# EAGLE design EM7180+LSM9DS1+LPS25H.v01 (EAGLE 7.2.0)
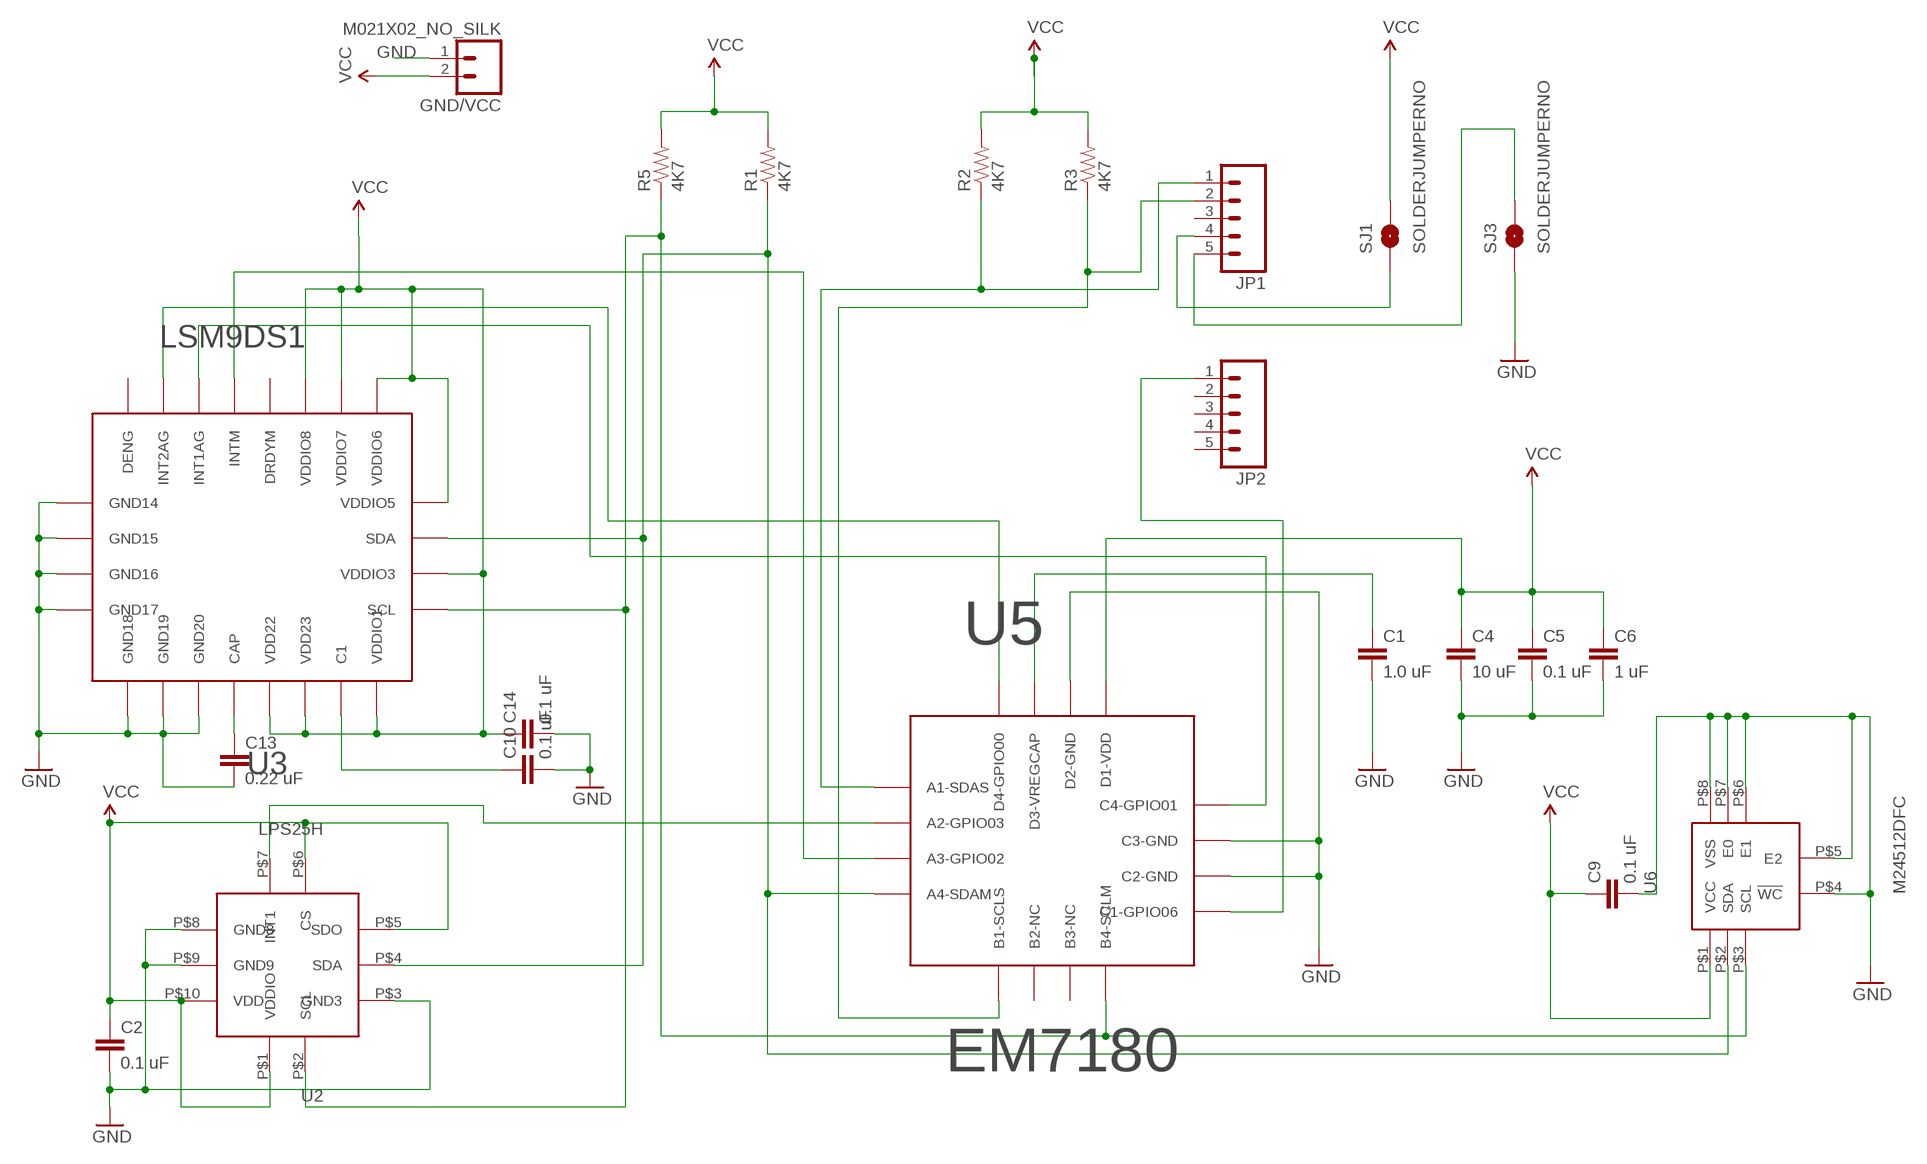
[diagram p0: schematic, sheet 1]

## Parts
C1  1.0 uF  CAP0402-CAP  [0402-CAP]
C2  0.1 uF  CAP0402-CAP  [0402-CAP]
C4  10 uF  CAP0402-CAP  [0402-CAP]
C5  0.1 uF  CAP0402-CAP  [0402-CAP]
C6  1 uF  CAP0402-CAP  [0402-CAP]
C9  0.1 uF  CAP0402-CAP  [0402-CAP]
C10  0.1 uF  CAP0402-CAP  [0402-CAP]
C13  0.22 uF  CAP0402-CAP  [0402-CAP]
C14  0.1 uF  CAP0402-CAP  [0402-CAP]
GND/VCC  M021X02_NO_SILK  [1X02_NO_SILK]
JP1  M05NO_SILK  [1X05_NO_SILK]
JP2  M05NO_SILK  [1X05_NO_SILK]
R1  4K7  0402RES.KW  [0402-RES]
R2  4K7  0402RES.KW  [0402-RES]
R3  4K7  0402RES.KW  [0402-RES]
R5  4K7  0402RES.KW  [0402-RES]
SJ1  SOLDERJUMPERNO  [SJ_2S-NO]
SJ3  SOLDERJUMPERNO  [SJ_2S-NO]
U2  LPS25H  [HCLGA-10L]
U3  LSM9DS1  [LGA-24LONG]
U5  EM7180  [WL-CSP16]
U6  M24512DFC  [M24512DFC]

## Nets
GND: C1.2 C2.2 C4.2 C5.2 C6.2 C9.2 C10.2 C13.2 C14.2 GND/VCC.1 SJ3.1 U2.P$3(GND3) U2.P$8(GND8) U2.P$9(GND9) U3.P$14(GND14) U3.P$15(GND15) U3.P$16(GND16) U3.P$17(GND17) U3.P$18(GND18) U3.P$19(GND19) U3.P$20(GND20) U5.P$10(C2-GND) U5.P$11(C3-GND) U5.P$14(D2-GND) U6.P$4(!WC) U6.P$5(E2) U6.P$6(E1) U6.P$7(E0) U6.P$8(VSS)
N$1: U2.P$7(INT1) U5.P$2(A2-GPIO03)
N$2: U3.P$10(INTM) U5.P$3(A3-GPIO02)
N$4: JP2.1 U5.P$9(C1-GPIO06)
N$5: U3.P$11(INT1AG) U5.P$12(C4-GPIO01)
N$6: U3.P$12(INT2AG) U5.P$16(D4-GPIO00)
N$7: JP1.4 SJ1.1
N$8: JP1.5 SJ3.2
N$9: C1.1 U5.P$15(D3-VREGCAP)
N$12: C13.1 U3.P$21(CAP)
N$14: C10.1 U3.P$24(C1)
SCL: R5.1 U2.P$2(SCL) U3.P$2(SCL) U5.P$8(B4-SCLM) U6.P$3(SCL)
SCL1: JP1.1 R2.1 U5.P$1(A1-SDAS)
SDA: R1.1 U2.P$4(SDA) U3.P$4(SDA) U5.P$4(A4-SDAM) U6.P$2(SDA)
SDA1: JP1.2 R3.1 U5.P$5(B1-SCLS)
VCC: C2.1 C4.1 C5.1 C6.1 C9.1 C14.1 GND/VCC.2 R1.2 R2.2 R3.2 R5.2 SJ1.2 U2.P$1(VDDIO) U2.P$5(SDO) U2.P$6(CS) U2.P$10(VDD) U3.P$1(VDDIO1) U3.P$3(VDDIO3) U3.P$5(VDDIO5) U3.P$6(VDDIO6) U3.P$7(VDDIO7) U3.P$8(VDDIO8) U3.P$22(VDD22) U3.P$23(VDD23) U5.P$13(D1-VDD) U6.P$1(VCC)
Unconnected: JP1.3 JP2.2 JP2.3 JP2.4 JP2.5 U3.P$9(DRDYM) U3.P$13(DENG) U5.P$6(B2-NC) U5.P$7(B3-NC)

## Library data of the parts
C1 C2 C4-C6 C9 C10 C13 C14 = SparkFun-Capacitors:CAP: Capacitor
GND/VCC = SparkFun-Connectors:M02: Standard 2-pin 0.1" header. Use with
JP1 JP2 = SparkFun-Connectors:M05: Header 5 Standard 5-pin 0.1" header. Use with straight break away headers (SKU : PRT-00116), right angle break away headers (PRT-00553), swiss pins (PRT-00743), machine pins (PRT-00117), and female headers (PRT-00115). Molex polarized connector foot print use with SKU : PRT-08230 with associated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
R1-R3 R5 = SparkFun-Resistors:0402RES.KW
SJ1 SJ3 = SparkFun-Retired:SOLDERJUMPER: Solder Jumper
U2 = Kris:LPS25H: HCLGA-10L package for the LPS25H ST pressure sensor
U3 = SparkFun-DigitalIC:LSM9DS1: LSM9DS1 3.0 mm x 3.5 mm 9-axis motion sensor by ST Microelectrinics in an LGA-24 device package
U5 = SparkFun-DigitalIC:EM7180: WL-CSP19 package for the EM7180 SENtral sensor fusion hub
U6 = Kris:M24512DFC: ST's M24512DFC6 512 Mbit EEPROM

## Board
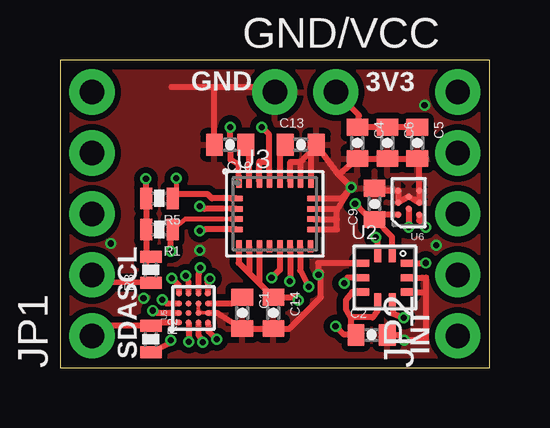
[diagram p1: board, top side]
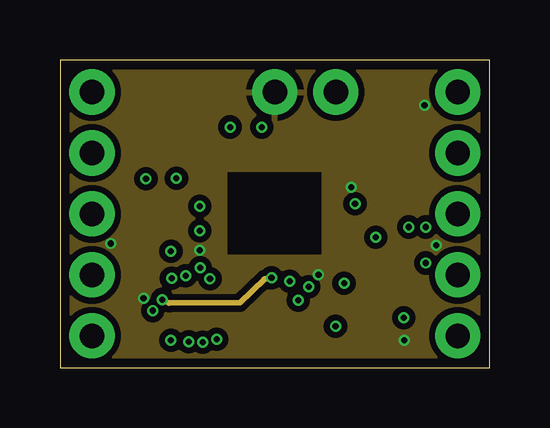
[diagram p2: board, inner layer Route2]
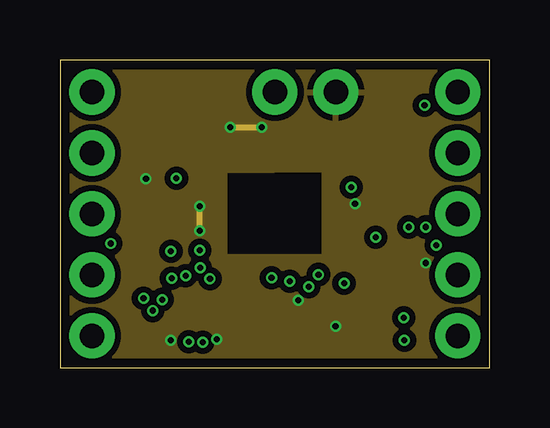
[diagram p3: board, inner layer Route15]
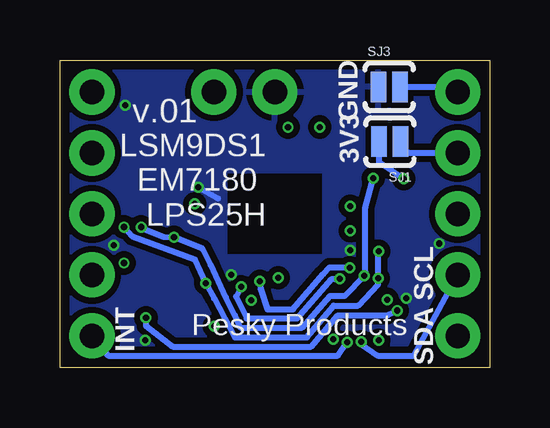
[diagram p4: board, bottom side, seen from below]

Size 17.91 x 12.83 mm. Coordinates in mm from the lower left corner, seen from the top.
Outline: 0,0 17.91,0 17.91,12.83 0,12.83 0,0
Copper layers (1*2*15*16): Top 0.035559375mm / dielectric 0.17018125mm / Route2 0.01778125mm / dielectric 47mil / Route15 0.01778125mm / dielectric 0.17018125mm / Bottom 0.035559375mm
Design rules "OSHPark-4layer *": minimum track width 5mil, minimum drill 10mil, track to track 5mil, track to pad 5mil, pad to pad 5mil, via to via 5mil, smd to smd 5mil, copper to edge 15mil, drill to drill 6mil, minimum pad ring 4mil, minimum via ring 4mil, stop-mask expansion 4mil, vias tented up to drill 20mil, thermal gap 10mil

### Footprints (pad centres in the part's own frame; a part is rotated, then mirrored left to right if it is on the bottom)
0402-CAP = smd 0.7 x 0.9: 1 -0.65,0; 2 0.65,0
1X02_NO_SILK = drill 1.016 pad 1.88: 1 0,0; 2 2.54,0
1X05_NO_SILK = drill 1.016 pad 1.88: 1 0,0; 2 2.54,0; 3 5.08,0; 4 7.62,0; 5 10.16,0
0402-RES = smd 0.5 x 0.9: 1 -0.55,0; 2 0.55,0
SJ_2S-NO = smd 0.635 x 1.27: 1 -0.45,0; 2 0.45,0
HCLGA-10L = smd 0.3 x 0.6: P$1 0.3,0.95; P$2 -0.3,0.95; P$6 -0.3,-0.95; P$7 0.3,-0.95 | smd 0.6 x 0.3: P$3 -0.95,0.6; P$4 -0.95,0; P$5 -0.95,-0.6; P$8 0.95,-0.6; P$9 0.95,0; P$10 0.95,0.6
LGA-24LONG = smd 0.23 x 0.5: P$1 -1.505,1.345; P$6 -1.505,-1.345; P$7 -1.075,-1.345; P$8 -0.645,-1.345; P$9 -0.22,-1.345; P$10 0.205,-1.345; P$11 0.63,-1.345; P$12 1.055,-1.345; P$13 1.48,-1.345; P$18 1.505,1.345; P$19 1.075,1.345; P$20 0.645,1.345; P$21 0.215,1.345; P$22 -0.215,1.345; P$23 -0.645,1.345; P$24 -1.075,1.345 | smd 0.5 x 0.23: P$2 -1.595,0.645; P$3 -1.595,0.215; P$4 -1.595,-0.215; P$5 -1.595,-0.645; P$14 1.595,-0.645; P$15 1.595,-0.215; P$16 1.595,0.215; P$17 1.595,0.645
WL-CSP16 = smd 0.24 x 0.24: P$1 -0.6,0.6; P$2 -0.2,0.6; P$3 0.2,0.6; P$4 0.6,0.6; P$5 -0.6,0.2; P$6 -0.2,0.2; P$7 0.2,0.2; P$8 0.6,0.2; P$9 -0.6,-0.2; P$10 -0.2,-0.2; P$11 0.2,-0.2; P$12 0.6,-0.2; P$13 -0.6,-0.6; P$14 -0.2,-0.6; P$15 0.2,-0.6; P$16 0.6,-0.6
M24512DFC = smd 0.27 x 0.27: P$1 0.433,0.5; P$2 -0.433,0.5; P$3 0,0.25; P$4 0.433,0; P$5 -0.433,0; P$6 0,-0.25; P$7 0.433,-0.5; P$8 -0.433,-0.5

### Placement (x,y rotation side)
C1  7.59,2.29 270 top
C2  12.98,1.37 0 top
C4  12.39,9.37 270 top
C5  14.88,9.37 270 top
C6  13.64,9.37 270 top
C9  13.11,6.83 90 top
C10  7.09,9.3 180 top
C13  10.03,9.3 0 top
C14  8.89,2.29 270 top
GND/VCC  8.95,11.49 0 top
JP1  1.33,1.33 90 top
JP2  16.57,1.33 90 top
R1  4.14,5.77 180 top
R2  3.78,1.19 270 top
R3  3.78,4.09 90 top
R5  4.14,7.06 180 top
SJ1  4.17,9.42 180 bottom
SJ3  4.19,11.71 0 bottom
U2  13.54,3.76 0 top
U3  8.95,6.41 0 top
U5  5.56,2.49 90 top
U6  14.53,6.88 180 top

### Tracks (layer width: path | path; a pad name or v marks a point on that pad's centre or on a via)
GND  (via drill 0.25)
  Top 0.152: U5.P$11 U5.P$10 U5.P$14
  Top 0.254: SJ3.1 6.38,11.71 | 6.38,11.71 8.74,11.71 GND/VCC.1 | U5.P$14 6.56,2.29 C1.2 C14.2 9.56,1.64 10.87,2.95 10.87,3.99 v10.77,3.89 10.76,4.36 U2.P$3 | U3.P$19 10.03,8.59 | 10.03,8.59 C13.2 | U3.P$20 9.6,8.13 9.6,8.59 10.03,8.59 | C2.2 14.07,1.37 v14.35,1.14 15.16,1.14 15.24,1.22 15.24,3.12 | U3.P$17 11.76,7.06 v12.14,7.52 | U3.P$14 11.53,5.77 11.53,6.17 | 11.53,6.17 11.53,6.55 | 11.53,6.55 12.09,7.47 v12.14,7.52 | U3.P$16 11.46,6.63 11.53,6.55 | U3.P$15 11.51,6.2 11.53,6.17 | U3.P$18 10.46,8.89 C13.2 | v12.14,7.52 11.58,8.09 | 11.58,8.09 C13.2 | 11.58,8.09 11.66,8.09 C4.2 C6.2 C5.2 14.96,8.85 U6.P$8 U6.P$5 14.76,7.01 U6.P$6 14.32,7.01 U6.P$4 U6.P$7 13.21,7.38 C9.2 | U2.P$9 15.24,3.76 15.24,3.12 | U2.P$8 15.21,3.16 15.24,3.12 | C10.2 6.44,11.65 6.38,11.71
  Bottom 0.254: v12.14,7.52 11.33,7.06
  other vias: 15.19,10.95 2.11,5.18 5.82,4.9 15.67,5.11 3.48,2.9
  pour Bottom (isolate 0.254): 0,12.83 17.91,12.83 17.91,0 11,0 11,8.18 6.91,8.18 6.91,4.67 10.92,4.67 10.92,0 0.03,0
  pour Route2 (isolate 0.254): 0,12.83 17.91,12.83 17.91,0 10.97,0 10.97,8.2 6.91,8.23 6.91,4.67 10.87,4.65 10.87,0 0.03,0
  pour Top (isolate 0.254): 0,12.83 17.86,12.83 17.86,0 14.83,0 14.83,5.08 12.24,5.08 12.24,2.46 14.76,2.46 14.76,0 10.9,0 10.95,8.15 6.91,8.15 6.93,4.67 10.82,4.67 10.82,0 -0.03,0 -0.03,12.8
N$1  (via drill 0.25)
  Top 0.254: U2.P$7 13.86,2.27 v14.33,2.08 | v3.86,2.39 4.05,2.29 U5.P$2
  Bottom 0.254: v14.33,2.08 14.33,1.75 13.21,0.89 7.44,0.89 6.33,2.18 4.27,2.18 v3.86,2.39
N$2  (via drill 0.25)
  Top 0.254: U3.P$10 9.16,4.08 v8.81,3.76 | v4.27,2.85 4.41,2.69 U5.P$3
  Route2 0.254: v8.81,3.76 8.51,3.68 7.49,2.72 4.55,2.69 v4.27,2.85
N$4  (via drill 0.25)
  Top 0.254: U5.P$9 5.76,1.38 v5.94,1.07
  Bottom 0.254: JP2.1 15.9,0.51 6.33,0.51 v5.94,1.07
N$5  (via drill 0.25)
  Top 0.254: U3.P$11 9.58,3.64 v9.58,3.61 | v5.84,4.17 5.77,3.86 U5.P$12
  Bottom 0.254: v9.58,3.61 9.55,3.28 9.27,2.44 8.2,2.44 6.93,3.91 6.68,4.19 5.92,4.19 v5.84,4.17
N$6  (via drill 0.25)
  Top 0.254: U3.P$12 10.01,4.06 v10.36,3.38 | v6.25,3.71 6.15,3.56 6.15,3.1 U5.P$16
  Bottom 0.254: v10.36,3.38 10.57,2.97 10.13,2.06 8.03,2.06 6.58,3.71 v6.25,3.71
N$7
  Bottom 0.152: 3.76,9.04 SJ1.1
  Bottom 0.254: 3.76,9.04 3.79,9.09 3.38,8.97 1.88,8.97 JP1.4
N$8
  Bottom 0.254: 3.68,12.22 SJ3.2 1.55,11.71 JP1.5
N$9
  Top 0.254: U5.P$15 7.15,2.69 C1.1
N$12
  Top 0.254: U3.P$21 9.17,9 C13.1
N$14
  Top 0.254: U3.P$24 7.88,8.9 C10.1
SCL  (via drill 0.25)
  Top 0.203: v4.85,7.9 4.85,7.48 R5.1
  Top 0.254: U5.P$8 5.36,3.58 v5.23,3.83 | R5.1 4.87,7.24 6.15,7.24 6.33,7.06 U3.P$2 | U2.P$2 13.24,5.05 13.23,5.28 13.18,5.41 v13.16,5.44 | U6.P$3 v14.53,5.87
  Bottom 0.254: v4.85,7.9 5.18,6.68 5.18,3.99 v5.23,3.83 6.04,3 6.66,3 7.82,1.68 10.39,1.68 10.62,2.18 11,2.92 11.63,4.29 11.96,4.95 v13.16,5.44 13.59,5.46 14.38,5.77 v14.53,5.87
SCL1
  Top 0.254: JP1.1 1.79,1.74 R2.1 4.05,1.89 U5.P$1
SDA  (via drill 0.25)
  Top 0.203: U3.P$4 5.22,6.2 R1.1
  Top 0.254: U5.P$4 4.96,3.42 v4.65,3.73 | v4.62,4.85 4.62,5.6 R1.1 | U2.P$4 11.99,3.76 v11.84,3.53 | U6.P$2 14.96,6.15 v15.24,5.87
  Bottom 0.254: v4.62,4.85 4.65,4.62 v4.65,3.73 4.65,3.48 5.49,2.59 6.5,2.59 7.62,1.27 10.62,1.27 11.48,2.9 v11.84,3.53 12.29,4.52 14.9,5.49 v15.24,5.87
SDA1  (via drill 0.25)
  Top 0.254: R3.1 2.15,3.56 JP1.2 | U5.P$5 v5.36,1.09
  Bottom 0.254: v5.36,1.09 5.36,0.99 4.67,0.51 3.17,0.51 JP1.2
VCC  (via drill 0.25)
  Top 0.254: C5.1 C6.1 C4.1 12.46,10.52 GND/VCC.2 10.79,11.48 | U6.P$1 13.23,6.38 C9.1 | v3.58,7.87 3.58,7.59 R5.2 R1.2 3.59,4.35 R3.2 | R2.2 4.55,1.02 v4.62,1.14 | U5.P$13 6.19,1.51 v6.53,1.19 | C9.1 13.08,6.02 v12.29,6.83 | U3.P$6 7.45,4.38 | U2.P$1 13.84,5.45 C9.1 | U2.P$6 13.24,2.39 13.03,2.11 12.14,2.11 12.12,2.06 | U2.P$5 12.18,3.16 11.91,2.82 11.91,2.44 12.12,2.06 | U2.P$10 v15.23,4.36 v15.24,4.37 | v11.48,1.73 11.83,1.38 12.12,1.38 C2.1 12.12,1.58 12.12,2.06 | U3.P$22 8.71,8.63 | U3.P$23 8.31,8.59 8.67,8.59 8.71,8.63 | U3.P$1 7.45,8 7.44,8.46 7.11,8.66 v7.09,10.03 | U3.P$5 6.05,5.77 v5.82,5.71 | U3.P$7 7.88,3.95 | U3.P$8 8.31,3.52 | 7.45,4.38 7.88,3.95 | 7.44,4.37 7.45,4.38 | U3.P$3 6.02,6.63 v5.82,6.73 | v9.93,2.82 9.84,2.94 C14.1 8.31,3.52 | 7.88,3.95 8.31,3.52 | 8.71,8.63 8.71,9.73 v8.41,10.03
  Route15 0.254: v6.53,1.19 6.5,1.19 | 5.79,6.73 v5.82,6.73 v5.82,5.71 | v11.48,1.73 11.46,1.75 | v7.09,10.03 v8.41,10.03 | v9.93,2.82 9.98,2.77
  Bottom 0.254: SJ1.2 4.62,8.76 4.62,8.59 4.27,8.36 v3.58,7.87
  pour Route15 (isolate 0.254): 0,12.83 17.91,12.83 17.91,0 10.97,0.03 10.97,8.2 6.91,8.18 6.91,4.67 10.9,4.67 10.9,0 0.03,0

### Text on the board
tPlace: GND | 3V3 | SCL | INT | SDA
bPlace: GND | 3V3 | v.01 | LSM9DS1 / EM7180 / LPS25H | SCL | SDA | INT | Pesky Products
